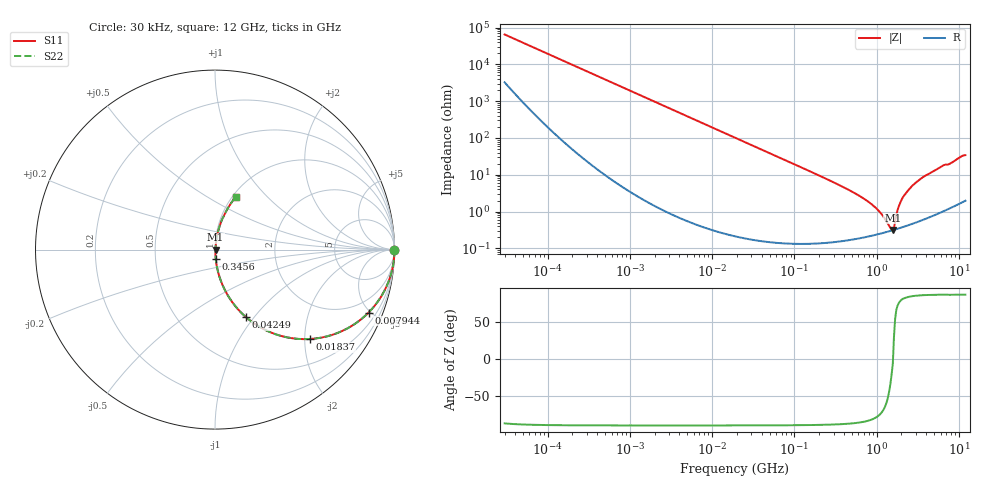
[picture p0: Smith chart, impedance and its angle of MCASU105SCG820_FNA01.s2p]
! MCASU105SCG820_FNA01  S-PARAMETER MODEL  ( General Type )
! Model Generated by TAIYO YUDEN Corporation (http://www.ty-top.com)
! Version 1.0
! TAIYO YUDEN Control No. 130207
! Copyright(c) 2013 TAIYO YUDEN CO.,LTD. All Rights Reserved.
! Product Description (link to TY-COMPAS)
! https://ds.yuden.co.jp/TYCOMPAS/or/detail?pn=MCASU105SCG820JFNA01&u=M
! Products Name : Multilayer Ceramic Capacitors
! Characteristics :
!  Capacitance : 82 pF , Rated Voltage : 50V , TCC : CG / C0G
!  Case Size : 1.0 x 0.5 / 0.039 x 0.02 [mm/inch] , Thickness : 0.5 / 0.02 [mm/inch]
!  (Conditions: Temperature = 25 degC , DC Bias Current/Voltage = 0A / 0V)
! External Node Assignments :
!  1  o---| |---o  2
! GND o---------o GND
! Frequency Range : 30000Hz  -  12GHz  [ 401 STEP ]
# MHz S RI R 50
! Freq[MHz].  S11 Real  S11 Imag  S21 Real  S21 Imag  S12 Real  S12 Imag  S22 Real  S22 Imag
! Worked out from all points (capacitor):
!   401 points, 30 kHz to 12 GHz, reference 50 ohm
!   read as one part in series: C = 82.1 pF near 32 kHz
!   lowest |Z| = 314 mohm at 1.573 GHz (marker M1)
!   series resonance near 1.582 GHz, so ESL is about 120 pH
!   S11 on the Smith chart (normalised r, x): 30 kHz: open; 7.944 MHz: 1.01, -4.88; 18.37 MHz: 1.00, -2.11; 42.49 MHz: 1.00, -0.91; 345.6 MHz: 1.00, -0.11; 12 GHz: 1.04, +0.68
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0.03  0.9999 -0.00154  7.98e-05 0.00154  7.98e-05 0.00154  0.9999 -0.00154
0.260295  0.9998 -0.0134  0.000234 0.0134  0.000234 0.0134  0.9998 -0.0134
2.258455  0.9864 -0.1149  0.0136 0.1149  0.0136 0.1149  0.9864 -0.1149
7.943506  0.8558 -0.3505  0.1442 0.3505  0.1442 0.3505  0.8558 -0.3505
18.37156  0.5266 -0.4983  0.4734 0.4983  0.4734 0.4983  0.5266 -0.4983
18.97367  0.5106 -0.4988  0.4894 0.4988  0.4894 0.4988  0.5106 -0.4988
42.48934  0.1729 -0.3765  0.8271 0.3765  0.8271 0.3765  0.1729 -0.3765
75.92288  0.0621 -0.2386  0.9379 0.2386  0.9379 0.2386  0.0621 -0.2386
164.6252  0.0147 -0.1146  0.9853 0.1146  0.9853 0.1146  0.0147 -0.1146
345.6326  0.00436 -0.0531  0.9956 0.0531  0.9956 0.0531  0.00436 -0.0531
880.5704  0.00245 -0.0152  0.9976 0.0152  0.9976 0.0152  0.00245 -0.0152
1139.739  0.00262 -0.00829  0.9974 0.00829  0.9974 0.00829  0.00262 -0.00829
1428.372  0.00293 -0.00269  0.9971 0.00269  0.9971 0.00269  0.00293 -0.00269
1523.532  0.00305 -0.00113  0.997 0.00113  0.997 0.00113  0.00305 -0.00113
1573.464  0.00311 -0.000358  0.9969 0.000358  0.9969 0.000358  0.00311 -0.000358
1848.769  0.00364 0.0128  0.9964 -0.0128  0.9964 -0.0128  0.00364 0.0128
1971.936  0.00398 0.0186  0.996 -0.0186  0.996 -0.0186  0.00398 0.0186
2243.435  0.00488 0.0297  0.9951 -0.0297  0.9951 -0.0297  0.00488 0.0297
2722.352  0.00715 0.05  0.9928 -0.05  0.9928 -0.05  0.00715 0.05
3758.338  0.0138 0.0872  0.9862 -0.0872  0.9862 -0.0872  0.0138 0.0872
6096.395  0.0355 0.1585  0.9645 -0.1585  0.9645 -0.1585  0.0355 0.1585
12000  0.1178 0.2948  0.8822 -0.2948  0.8822 -0.2948  0.1178 0.2948
